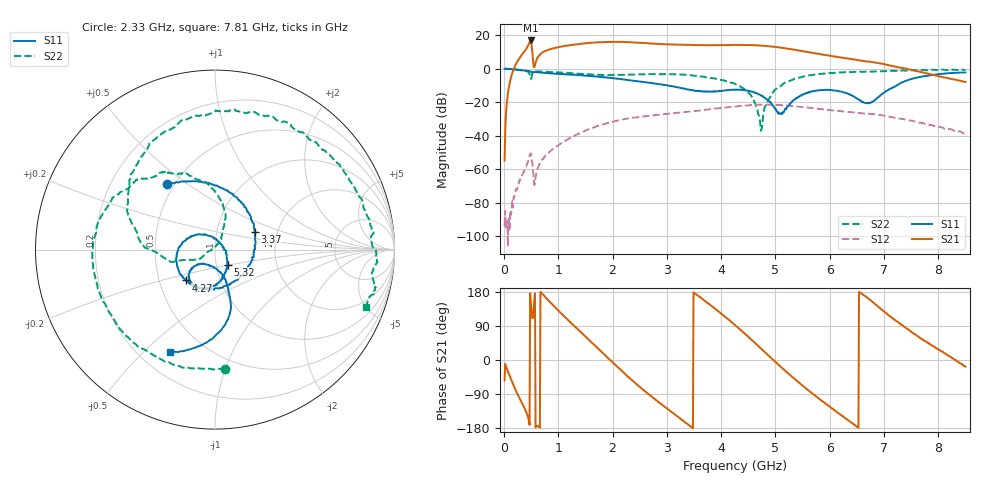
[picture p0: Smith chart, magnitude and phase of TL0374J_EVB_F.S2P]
!Agilent Technologies,E5071C,MY46523237,B.13.01
!Date: Sat Oct 07 10:37:43 2023
!Data & Calibration Information:
!Freq	S11:SOLT2(ON)	S21:SOLT2(ON)	S12:SOLT2(ON)	S22:SOLT2(ON)
!PortZ  Port1:50+j0  Port2:50+j0
!Above PortZ is port z conversion or system Z0 setting when saving the data.
!When reading, reference impedance value at option line is always used.
# Hz S dB R 50
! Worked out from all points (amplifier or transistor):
!   850 points, 10 MHz to 8.5 GHz, reference 50 ohm
!   highest |S21| = 16.9 dB at 490 MHz (marker M1)
!   |S21| within 3 dB of that: 1.18 GHz to 4.708 GHz (3.528 GHz wide, 120 % of centre)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
!   unconditionally stable (mu >= 1): 16.17 MHz to end of sweep
!   at 1.42 GHz: K = 2.55, MAG = 19.6 dB, |S12| = -38.1 dB
!   at 4.26 GHz: K = 1.31, MAG = 15.0 dB, |S12| = -22.5 dB
!   at 8.5 GHz: K = 7.66, MAG = 3.6 dB, |S12| = -38.8 dB
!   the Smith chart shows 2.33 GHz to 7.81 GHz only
!   S11 on the Smith chart (normalised r, x): 2.33 GHz: 0.46, +0.42; 3.37 GHz: 1.53, +0.33; 4.27 GHz: 0.68, -0.25; 5.32 GHz: 1.13, -0.20; 7.81 GHz: 0.32, -0.60
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1e7  -0.07 -1.8  -54.76 -53.6  -93.87 144.8  0.04 -4.3
2.3e8  -0.55 -33.1  3.50 -84.3  -72.50 175.4  -0.55 -88.1
4e8  -1.19 -55.4  11.40 -134.1  -58.71 151.5  -1.33 -137.7
4.6e8  -1.40 -63.3  15.16 -162.1  -53.28 132.9  -2.49 -156.8
4.9e8  -1.77 -67.8  16.86 158.6  -50.55 92.2  -5.84 -157.1
5.6e8  -2.01 -72.0  1.09 163.5  -69.38 81.7  -1.74 -154.1
9.1e8  -2.89 -108.6  12.19 143.3  -47.73 109.6  -2.12 143.3
1.43e9  -3.99 -158.1  14.85 71.5  -37.97 53.3  -3.05 68.0
1.9e9  -5.29 160.4  16.00 7.4  -32.50 -1.4  -3.79 -12.2
2.33e9  -6.91 126.1  15.77 -50.0  -29.49 -53.3  -3.48 -85.1
2.84e9  -9.15 85.2  14.78 -110.3  -27.56 -108.7  -3.28 -150.0
3.37e9  -12.28 24.3  14.32 -167.8  -25.64 -161.2  -3.72 160.4
3.81e9  -13.55 -53.8  14.01 144.0  -24.10 155.1  -5.54 126.1
4.26e9  -12.49 -131.8  14.22 91.7  -22.50 106.4  -9.10 93.4
4.27e9  -12.52 -133.5  14.18 90.2  -22.46 105.2  -9.34 93.2
4.81e9  -17.62 140.5  13.59 20.1  -21.47 39.3  -22.67 -151.0
5.32e9  -19.15 -50.5  11.48 -46.0  -22.31 -22.3  -6.53 164.3
5.67e9  -13.47 -95.1  9.52 -87.0  -23.50 -60.4  -3.81 131.8
6.31e9  -14.63 -139.0  6.29 -155.6  -25.69 -124.9  -2.16 78.3
7.09e9  -12.48 -72.0  2.11 117.6  -28.63 152.6  -1.39 22.7
7.81e9  -4.08 -113.8  -2.95 44.9  -33.43 83.6  -0.89 -20.7
8.5e9  -2.20 -163.5  -7.91 -17.6  -38.83 21.4  -0.78 -54.1
